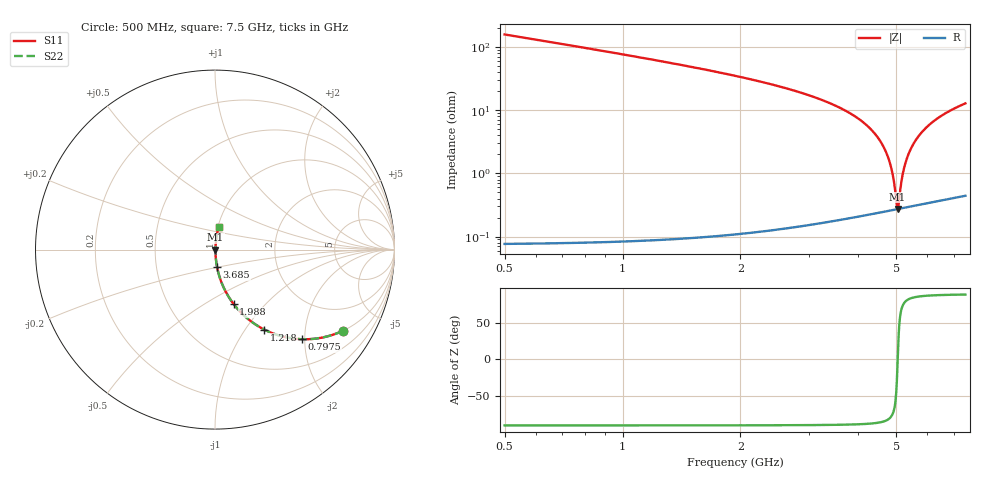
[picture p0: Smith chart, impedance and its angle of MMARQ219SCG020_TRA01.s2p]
! MMARQ219SCG020_TRA01  S-PARAMETER MODEL  ( General Type )
! Model Generated by TAIYO YUDEN Corporation (http://www.ty-top.com)
! Version 1.0
! TAIYO YUDEN Control No. 180601
! Copyright(c) 2018 TAIYO YUDEN CO.,LTD. All Rights Reserved.
! Product Description (link to TY-COMPAS)
! https://ds.yuden.co.jp/TYCOMPAS/or/detail?pn=MMARQ219SCG020BTRA01&u=M
! Products Name : Multilayer Ceramic Capacitors
! Characteristics :
!  Capacitance : 2 pF , Rated Voltage : 250V , TCC : CG / C0G
!  Case Size : 2.0 x 1.25 / 0.079 x 0.049 [mm/inch] , Thickness : 0.85 / 0.033 [mm/inch]
!  (Conditions: Temperature = 25 degC , DC Bias Current/Voltage = 0A / 0V)
! External Node Assignments :
!  1  o---| |---o  2
! GND o---------o GND
! Frequency Range : 500MHz  -  7500MHz  [ 401 STEP ]
# MHz S RI R 50
! Freq[MHz].  S11 Real  S11 Imag  S21 Real  S21 Imag  S12 Real  S12 Imag  S22 Real  S22 Imag
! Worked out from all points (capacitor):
!   401 points, 500 MHz to 7.5 GHz, reference 50 ohm
!   read as one part in series: C = 2 pF near 535 MHz
!   lowest |Z| = 274 mohm at 5.032 GHz (marker M1)
!   series resonance near 5.038 GHz, so ESL is about 500 pH
!   S11 on the Smith chart (normalised r, x): 500 MHz: 1.00, -3.15; 797.5 MHz: 1.00, -1.95; 1.218 GHz: 1.00, -1.23; 1.988 GHz: 1.00, -0.68; 3.685 GHz: 1.00, -0.20; 7.5 GHz: 1.01, +0.26
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500  0.7129 -0.4522  0.2871 0.4522  0.2871 0.4522  0.7129 -0.4522
797.5  0.4863 -0.4994  0.5137 0.4994  0.5137 0.4994  0.4863 -0.4994
1217.5  0.275 -0.4458  0.725 0.4458  0.725 0.4458  0.275 -0.4458
1672.5  0.1525 -0.3583  0.8475 0.3583  0.8475 0.3583  0.1525 -0.3583
1987.5  0.1032 -0.3027  0.8968 0.3027  0.8968 0.3027  0.1032 -0.3027
2845  0.0362 -0.1831  0.9638 0.1831  0.9638 0.1831  0.0362 -0.1831
3685  0.0118 -0.0988  0.9882 0.0988  0.9882 0.0988  0.0118 -0.0988
4000  0.00738 -0.0726  0.9926 0.0726  0.9926 0.0726  0.00738 -0.0726
4420  0.00401 -0.0411  0.996 0.0411  0.996 0.0411  0.00401 -0.0411
4700  0.00297 -0.0218  0.997 0.0218  0.997 0.0218  0.00297 -0.0218
4875  0.00272 -0.0103  0.9973 0.0103  0.9973 0.0103  0.00272 -0.0103
4927.5  0.00269 -0.00695  0.9973 0.00695  0.9973 0.00695  0.00269 -0.00695
4997.5  0.0027 -0.00254  0.9973 0.00254  0.9973 0.00254  0.0027 -0.00254
5032.5  0.00271 -0.000354  0.9973 0.000354  0.9973 0.000354  0.00271 -0.000354
5067.5  0.00274 0.00181  0.9973 -0.00181  0.9973 -0.00181  0.00274 0.00181
5172.5  0.00287 0.00823  0.9971 -0.00823  0.9971 -0.00823  0.00287 0.00823
5242.5  0.00301 0.0124  0.997 -0.0124  0.997 -0.0124  0.00301 0.0124
5330  0.00322 0.0176  0.9968 -0.0176  0.9968 -0.0176  0.00322 0.0176
5557.5  0.00401 0.0307  0.996 -0.0307  0.996 -0.0307  0.00401 0.0307
5890  0.00569 0.0488  0.9943 -0.0488  0.9943 -0.0488  0.00569 0.0488
6345  0.00885 0.0721  0.9911 -0.0721  0.9911 -0.0721  0.00885 0.0721
7500  0.0203 0.1248  0.9797 -0.1248  0.9797 -0.1248  0.0203 0.1248
